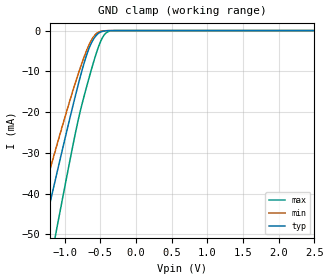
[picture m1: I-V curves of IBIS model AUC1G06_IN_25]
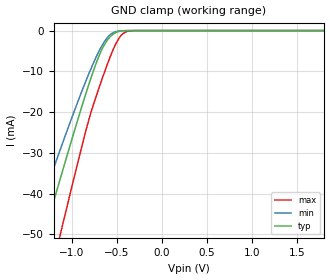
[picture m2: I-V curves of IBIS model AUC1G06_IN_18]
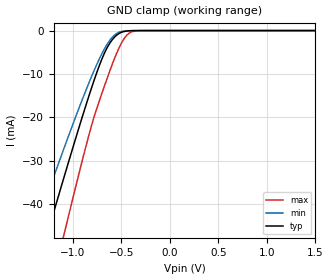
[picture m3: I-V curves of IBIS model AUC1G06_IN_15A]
| TEXAS INSTRUMENTS INCORPORATED
| Standard Linear and Logic Group
| IBIS Model of SN74AUC1G06
| Single Inverter Buffer/Driver with Open-Drain Output
| This file contains package information for the following:
|  SOT 5-pin (DCK) package as [Component] AUC1G06_DCK
|  SOT 5-pin (DBV) package as [Component] AUC1G06_DBV
|  NanoStar WCSP 5-pin (YEA) package as [Component] AUC1G06_YEA
|  NanoFree WCSP 5-pin (YZA) package as [Component] AUC1G06_YZA
| This device can be powered at the following Vccs:
|  2.5 volt Vcc
|  1.8 volt Vcc
|  1.5 volt Vcc
|  1.2 volt Vcc
|  0.8 volt Vcc
| This file provides unique models under the [Model Selector] for each Vcc.
| For operation at a specific Vcc, select the appropriate model after each
| [Model Selector] keyword.
[IBIS Ver]   3.2
[Comment char]  |_char
[File Name]   sn74auc1g06.ibs
[File Rev]   1.1 | x_die
[Date]   March 1, 2003
[Source]   Data created from TI-SPICE simulations at TI-SLL.
[Notes]   The following is an IBIS list for the AUC1G06.
   Please contact sllibis@ti.com with questions and
   comments concerning SLL IBIS models.
   - The slow Rising Waveforms in the AUC1G06_OUT are normal for
   this open-drain (TPLZ) device.
   - The SN74AUC1G06 has output feedback control circuitry.
   This will cause some non-monotonicity warnings.
   - The SN74AUC1G06 inputs has no power clamp diode.
   Therefore, the input power clamp data are not included.
   - The SN74AUC1G06 outputs has no power clamp diode.
   Therefore, the output power clamp data are not included.
[Disclaimer] Property of Texas Instruments Incorporated.  Unauthorized
   reproduction and/or distribution is strictly prohibited.
   This product is protected under copyright law.
   Created  2002, (C) Copyright  2002, Texas Instruments
   Incorporated, All Rights Reserved
   UNLESS THERE IS A SIGNED, WRITTEN AGREEMENT TO THE
   CONTRARY, TEXAS INSTRUMENTS (TI) IS PROVIDING THE IBIS
   MODELS  AND WITHOUT ANY WARRANTY, EXPRESSED OR
   IMPLIED.  TI assumes no liability for:
   1) the accuracy of the IBIS models provided to your
   company;
   2) the proper functioning of these IBIS Models in your
   design or for any resulting applications; or
   3) infringement of patents, copyrights or intellectual
   property rights resulting from your use of these IBIS
   models.
   TI provides IBIS Models as a service to our customers.
   You and your company shall not distribute, sell or give
   these models to anyone else without prior written
   permission from TI.
   TI reserves the right to make changes to our products or
   to discontinue any semiconductor product or service
   without notice, and advises our customers to obtain the
   latest version of relevant information to verify, before
   placing orders, that the information being relied on is
   current.
   Please be aware that your receipt and use of the IBIS
   information provided shall serve as acceptance of these
   terms and conditions.  If you do not accept these terms,
   you should return or destroy the IBIS models and any
   other accompanying information immediately.
| Component AUC1G06_DCK 5-pin SOT
[Component]   AUC1G06_DCK
[Manufacturer]   Texas Instruments, Inc.
[Package]
|   typ   min   max
R_pkg   2.000e-02   1.700e-02   2.500e-02
L_pkg   9.980e-10   8.810e-10   1.069e-09
C_pkg   1.460e-13   1.180e-13   2.050e-13
[Pin]   signal_name   model_name   R_pin   L_pin   C_pin
1   NC   NC   1.900e-02   1.069e-09   1.620e-13
2   A   AUC1G06_IN   1.800e-02   8.810e-10   1.210e-13
3   GND   GND   1.700e-02   1.031e-09   2.050e-13
4   Y   AUC1G06_OUT   2.000e-02   9.600e-10   1.240e-13
5   VCC   POWER   2.500e-02   1.049e-09   1.180e-13
| Component AUC1G06_DBV 5-pin SOT
[Component]   AUC1G06_DBV
[Manufacturer]   Texas Instruments, Inc.
[Package]
|   typ   min   max
R_pkg   2.500e-02   2.100e-02   2.900e-02
L_pkg   1.529e-09   1.312e-09   1.906e-09
C_pkg   1.560e-13   1.100e-13   2.400e-13
[Pin]   signal_name   model_name   R_pin   L_pin   C_pin
1   NC   NC   2.100e-02   1.511e-09   1.440e-13
2   A   AUC1G06_IN   2.300e-02   1.312e-09   1.380e-13
3   GND   GND   2.900e-02   1.906e-09   2.400e-13
4   Y   AUC1G06_OUT   2.600e-02   1.541e-09   1.500e-13
5   VCC   POWER   2.500e-02   1.374e-09   1.100e-13
| Component AUC1G06_YEA 5-pin NanoStar WCSP
[Component]   AUC1G06_YEA
[Manufacturer]   Texas Instruments, Inc.
[Package]
|   typ   min   max
R_pkg   0.001   0.001   0.001
L_pkg   0.021nH   0.021nH   0.021nH
C_pkg   0.046pF   0.045pF   0.047pF
[Pin]   signal_name   model_name   R_pin   L_pin   C_pin
1   DNU   NC   0.001   0.021nH   0.046pF
2   A   AUC1G06_IN   0.001   0.021nH   0.047pF
3   GND   GND   0.001   0.021nH   0.046pF
4   Y   AUC1G06_OUT   0.001   0.021nH   0.045pF
5   VCC   POWER   0.001   0.021nH   0.045pF
| Component AUC1G06_YZA 5-pin NanoFree WCSP
[Component]   AUC1G06_YZA
[Manufacturer]   Texas Instruments, Inc.
[Package]
|   typ   min   max
R_pkg   0.001   0.001   0.001
L_pkg   0.021nH   0.021nH   0.021nH
C_pkg   0.046pF   0.045pF   0.047pF
[Pin]   signal_name   model_name   R_pin   L_pin   C_pin
1   DNU   NC   0.001   0.021nH   0.046pF
2   A   AUC1G06_IN   0.001   0.021nH   0.047pF
3   GND   GND   0.001   0.021nH   0.046pF
4   Y   AUC1G06_OUT   0.001   0.021nH   0.045pF
5   VCC   POWER   0.001   0.021nH   0.045pF
| Model AUC1G06_IN
[Model Selector]   AUC1G06_IN
AUC1G06_IN_25   2.5 volt Vcc
AUC1G06_IN_18   1.8 volt Vcc
AUC1G06_IN_15A   1.5 volt Vcc
AUC1G06_IN_12   1.2 volt Vcc
AUC1G06_IN_08   0.8 volt Vcc
| Model AUC1G06_OUT
[Model Selector]   AUC1G06_OUT
AUC1G06_OUT_25   2.5 volt Vcc
AUC1G06_OUT_18   1.8 volt Vcc
AUC1G06_OUT_15A   1.5 volt Vcc
AUC1G06_OUT_12   1.2 volt Vcc
AUC1G06_OUT_08   0.8 volt Vcc
| Models and submodels in the file (10): AUC1G06_IN_25 (Input), AUC1G06_IN_18 (Input), AUC1G06_IN_15A (Input), AUC1G06_IN_12 (Input), AUC1G06_IN_08 (Input), AUC1G06_OUT_25 (Open_drain), AUC1G06_OUT_18 (Open_drain), AUC1G06_OUT_15A (Open_drain), AUC1G06_OUT_12 (Open_drain), AUC1G06_OUT_08 (Open_drain)
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[Model]   AUC1G06_IN_25
Model_type  Input
Vinl=0.7
Vinh=1.7
| variable   typ   min   max
C_comp   2.25pF   1.86pF   2.74pF
[Temperature Range]   40   100   -40
| Ambient temperature   25   85   -40
[Voltage range]   2.5   2.3   2.7
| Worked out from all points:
|   GND clamp passes 1 mA (typ) near -0.55 V on its own axis
[GND Clamp]
| AUC1G06_IN_25
|   Voltage   I(typ)   I(min)   I(max)
-3.6V     -230.2mA   -193.8mA   -275.4mA
-1.465V   -62.46mA   -50.68mA   -81.32mA
-1.41V    -58.19mA   -47.14mA   -76.26mA
-1.3V     -49.69mA   -40.13mA   -66.14mA
-1.11V    -35.19mA   -28.25mA   -48.67mA
-845mV    -15.76mA   -12.61mA   -24.92mA
-720mV    -7.623mA   -6.181mA   -15.69mA
-625mV    -3.09mA    -2.403mA   -9.633mA
-515mV    -559.5uA   -308.9uA   -3.552mA
-430mV    -73.2uA    -35.77uA   -776.9uA
-325mV    -3.339uA   -2.035uA   -30.74uA
2.5V      313.9pA    402pA      470.4pA
[Model]   AUC1G06_IN_18
Model_type  Input
Vinl=0.5775
Vinh=1.2675
| variable   typ   min   max
C_comp   2.23pF   1.87pF   2.77pF
[Temperature Range]   40   100   -40
| Ambient temperature   25   85   -40
[Voltage range]   1.8   1.65   1.95
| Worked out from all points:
|   GND clamp passes 1 mA (typ) near -0.55 V on its own axis
[GND Clamp]
| AUC1G06_IN_18
|   Voltage   I(typ)   I(min)   I(max)
-3.6V     -230.2mA   -193.8mA   -275.4mA
-1.445V   -60.91mA   -49.39mA   -79.48mA
-1.29V    -48.93mA   -39.5mA    -65.22mA
-1.145V   -37.84mA   -30.41mA   -51.89mA
-1.1V     -34.44mA   -27.64mA   -47.76mA
-830mV    -14.72mA   -11.79mA   -23.67mA
-690mV    -5.96mA    -4.844mA   -13.74mA
-565mV    -1.381mA   -914.2uA   -6.102mA
-490mV    -326uA     -167.9uA   -2.495mA
-425mV    -63.97uA   -31.34uA   -688.8uA
-275mV    -662.6nA   -487.6nA   -4.372uA
1.8V      203.2pA    298.4pA    235.5pA
[Model]   AUC1G06_IN_15A
Model_type  Input
Vinl=0.49
Vinh=1.04
| variable   typ   min   max
C_comp   2.24pF   1.87pF   2.82pF
[Temperature Range]   40   100   -40
| Ambient temperature   25   85   -40
[Voltage range]   1.5   1.4   1.6
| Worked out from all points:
|   GND clamp passes 1 mA (typ) near -0.55 V on its own axis
[GND Clamp]
| AUC1G06_IN_15A
|   Voltage   I(typ)   I(min)   I(max)
-3.6V     -230.2mA   -193.8mA   -275.4mA
-1.39V    -56.64mA   -45.86mA   -74.42mA
-1.25V    -45.85mA   -36.97mA   -61.54mA
-1.095V   -34.06mA   -27.33mA   -47.3mA
-1.05V    -30.68mA   -24.59mA   -43.18mA
-810mV    -13.36mA   -10.7mA    -22.06mA
-685mV    -5.701mA   -4.633mA   -13.41mA
-565mV    -1.381mA   -914.2uA   -6.102mA
-490mV    -326uA     -167.9uA   -2.495mA
-425mV    -63.97uA   -31.34uA   -688.8uA
-280mV    -781.4nA   -563.5nA   -5.358uA
1.5V      165.9pA    259.7pA    172.1pA
